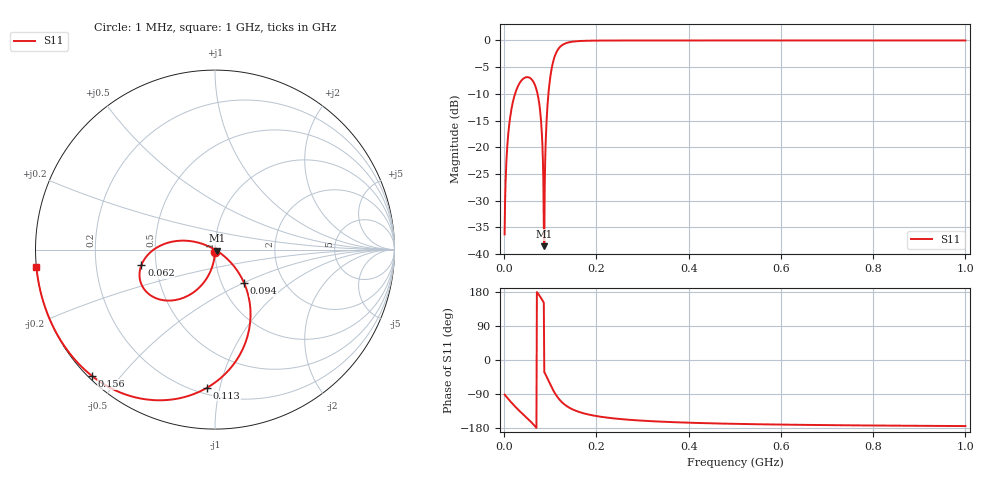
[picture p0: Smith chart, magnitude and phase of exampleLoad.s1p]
# MHz S RI R 50.0
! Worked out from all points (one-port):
!   999 points, 1 MHz to 1 GHz, reference 50 ohm
!   lowest |S11| = -38.5 dB at 87 MHz (marker M1), VSWR 1.02, Z = 51 - j0.649 ohm
!   |S11| at or under -10 dB: start of sweep to 23.59 MHz; 72.36 MHz to 95.97 MHz (23.61 MHz wide, 28 % of centre)
!   S11 on the Smith chart (normalised r, x): 1 MHz: 1.00, -0.03; 62 MHz: 0.41, -0.09; 94 MHz: 1.27, -0.51; 113 MHz: 0.24, -0.92; 156 MHz: 0.01, -0.42; 1 GHz: 0.00, -0.05
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1  -0.00039 -0.0153
8  -0.024 -0.1178
13  -0.0605 -0.1806
19  -0.1193 -0.2379
39  -0.3341 -0.2688
62  -0.41 -0.0862
70  -0.3475 -0.00463
76  -0.2547 0.0403
80  -0.1694 0.0499
84  -0.0691 0.0317
87  0.01 -0.00636
90  0.0847 -0.0683
92  0.1278 -0.1227
94  0.1623 -0.1863
97  0.1932 -0.2943
102  0.1812 -0.4827
113  -0.0436 -0.7692
126  -0.3424 -0.8386
139  -0.5383 -0.7918
156  -0.6856 -0.7038
192  -0.8271 -0.5547
251  -0.9107 -0.4111
376  -0.9633 -0.2678
502  -0.9799 -0.1989
626  -0.9872 -0.1589
751  -0.9912 -0.1322
876  -0.9935 -0.1132
1000  -0.995 -0.0991
